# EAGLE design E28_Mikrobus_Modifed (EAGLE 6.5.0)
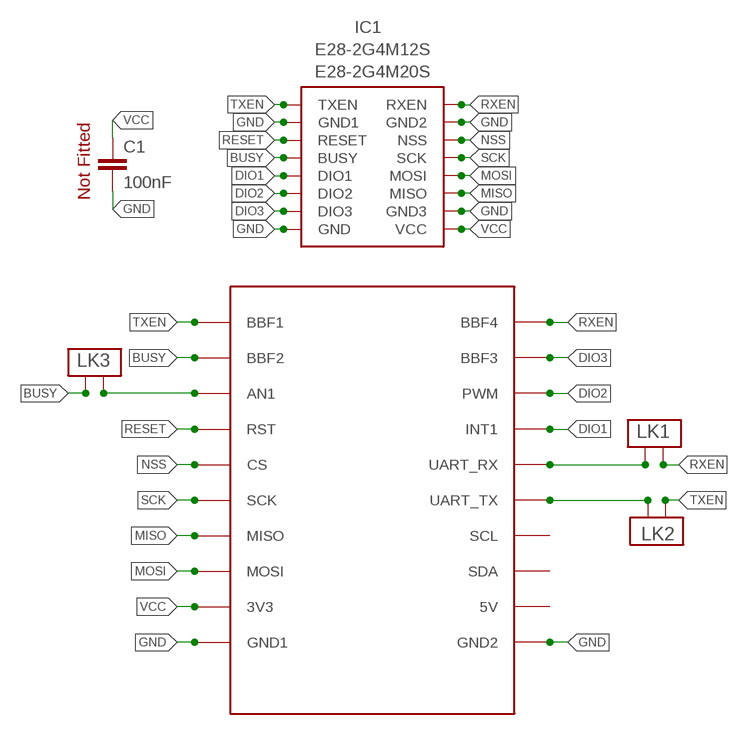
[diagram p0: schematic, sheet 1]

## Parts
C1  100nF  C-EUC0805  [C0805]
IC1  E28-2G4M12S  [E28-2G4M12S]
LK1  PCB_LINK  [PCB_LINK]
LK2  PCB_LINK  [PCB_LINK]
LK3  PCB_LINK  [PCB_LINK]
MB1  BBFRIENDY2  [PCB_SOCKET_BBFRIENDLY2]

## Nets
BUSY: IC1.BUSY LK3.P$2 MB1.BBF2
DIO1: IC1.DIO1 MB1.INT(INT1)
DIO2: IC1.DIO2 MB1.PWM
DIO3: IC1.DIO3 MB1.BBF3
GND [VDD]: C1.2 IC1.GND IC1.GND1 IC1.GND2 IC1.GND3 MB1.GND1(GND2) MB1.GND2(GND1)
MISO: IC1.MISO MB1.MISO
MOSI: IC1.MOSI MB1.MOSI
N$3: LK3.P$1 MB1.AN1
NSS: IC1.NSS MB1.CS
RESET: IC1.RESET MB1.RST
RXEN: IC1.RXEN LK1.P$1 MB1.BBF4
SCK: IC1.SCK MB1.SCK
TXEN: IC1.TXEN LK2.P$2 MB1.BBF1
UART_RX: LK1.P$2 MB1.RX(UART_RX)
UART_TX: LK2.P$1 MB1.TX(UART_TX)
VCC [VDD]: C1.1 IC1.VCC MB1.3V3
Unconnected: MB1.5V MB1.SCL MB1.SDA

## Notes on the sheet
- E28-2G4M20S
- Not Fitted

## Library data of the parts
C1 = resistor:C-EU: CAPACITOR, European symbol
IC1 = LMA2:E28-2G4M12S
LK1-LK3 = LMA2:PCB_LINK
MB1 = My_Mikrobus:BBFRIENDY2

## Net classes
0 default: width 0.152 mm
1 POWER: width 0.635 mm
2 VDD: width 0.635 mm

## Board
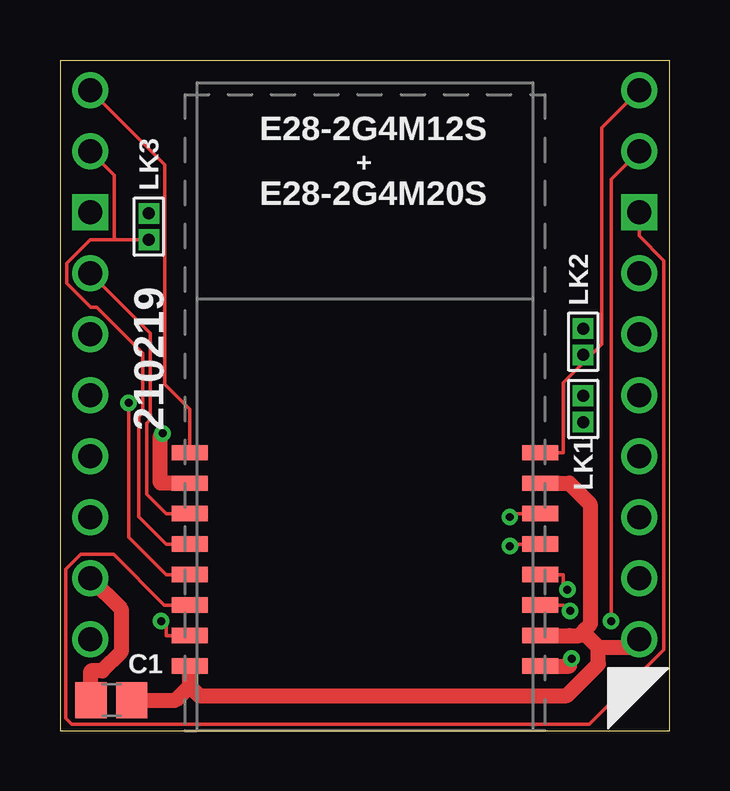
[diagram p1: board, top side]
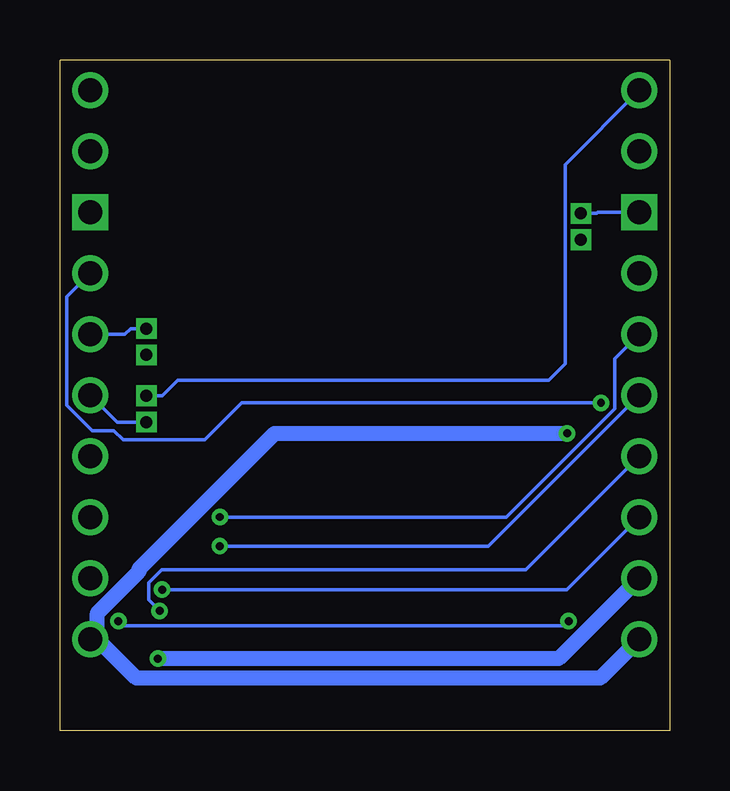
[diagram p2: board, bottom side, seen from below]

Size 25.4 x 27.94 mm. Coordinates in mm from the lower left corner, seen from the top.
Outline: 0,0 25.4,0 25.4,27.94 0,27.94 0,0
Copper layers (1*16): Top 0.0356mm / dielectric 1.5011mm / Bottom 0.0356mm
Design rules "LaenPCBOrder": minimum track width 6mil, minimum drill 13mil, track to track 6mil, track to pad 6mil, pad to pad 6mil, via to via 6mil, smd to smd 6mil, copper to edge 15mil, drill to drill 6mil, minimum pad ring 7mil, minimum via ring 7mil, stop-mask expansion 4mil, vias tented up to drill 0mil, thermal gap 10mil
tRestrict: area 4.6,15.4 to 20.9,28; area 6.5,1.9 to 19,15.4
bRestrict: area 4.6,15.4 to 20.9,27.9

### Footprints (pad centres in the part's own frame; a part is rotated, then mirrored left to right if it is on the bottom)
C0805 = smd 1.3 x 1.5: 1 -0.85,0; 2 0.85,0
E28-2G4M12S = smd 1.5 x 0.635: BUSY -7.3,7.77; DIO1 -7.3,6.5; DIO2 -7.3,5.23; DIO3 -7.3,3.96; GND -7.3,2.69; GND1 -7.3,10.31; GND2 7.3,10.31; GND3 7.3,3.96; MISO 7.3,5.23; MOSI 7.3,6.5; NSS 7.3,9.04; RESET -7.3,9.04; RXEN 7.3,11.58; SCK 7.3,7.77; TXEN -7.3,11.58; VCC 7.3,2.69
PCB_LINK = drill 0.5 pad 0.813 square: P$1 -0.55,0; P$2 0.55,0
PCB_SOCKET_BBFRIENDLY2 = drill 1: 3V3 -11.43,5.08; 5V 11.43,5.08; BBF1 -11.43,25.4; BBF2 -11.43,22.86; BBF3 11.43,22.86; BBF4 11.43,25.4; CS -11.43,15.24; GND1 -11.43,2.54; GND2 11.43,2.54; INT 11.43,17.78; MISO -11.43,10.16; MOSI -11.43,7.62; RST -11.43,17.78; RX 11.43,15.24; SCK -11.43,12.7; SCL 11.43,10.16; SDA 11.43,7.62; TX 11.43,12.7 | drill 1 square: AN1 -11.43,20.32; PWM 11.43,20.32

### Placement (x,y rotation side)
C1  2.14,1.27 0 top
IC1  12.7,0 0 top
LK1  21.8,16.2 90 top
LK2  21.8,13.4 90 top
LK3  3.7,21 270 top
MB1  12.7,1.27 0 top

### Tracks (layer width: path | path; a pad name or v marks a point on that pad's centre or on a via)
BUSY
  Top 0.152: IC1.BUSY 4.42,7.77 3.29,8.9 3.29,13.07 3.45,13.23 3.45,15.71 1.52,17.64 1.28,17.64 0.29,18.63 0.29,19.48 1.26,20.45 2.27,20.45 | 2.27,20.45 3.21,20.45 LK3.P$2 | MB1.BBF2 2.27,23.13 2.27,20.45
DIO1  (via drill 0.33 pad 0.69)
  Top 0.152: IC1.DIO1 4.42,6.5 2.86,8.06 v2.86,13.65
  Bottom 0.152: MB1.INT 25.11,18.07 25.11,13.55 24.05,12.5 23.15,12.5 22.77,12.12 19.36,12.12 17.83,13.65 v2.86,13.65
DIO2
  Top 0.152: MB1.PWM 24.13,20.61 25.16,19.58 25.16,3.37 22.06,0.27 0.49,0.27 0.24,0.51 0.24,6.71 0.86,7.34 2.24,7.34 4.35,5.23 IC1.DIO2
DIO3  (via drill 0.33 pad 0.69)
  Top 0.152: v22.97,4.56 22.97,22.97 MB1.BBF3 | v4.21,4.56 4.42,4.35 4.42,3.96 IC1.DIO3
  Bottom 0.152: v4.21,4.56 4.41,4.37 22.77,4.37 v22.97,4.56
GND  (via drill 0.33 pad 0.69)
  Top 0.635: 21.79,4.11 22.43,3.47 | 21.79,4.11 22.09,4.41 22.09,9.44 21.22,10.31 IC1.GND2 | 21.79,4.11 21.64,3.96 21.22,3.96 IC1.GND3 | 5.4,1.85 5.8,1.46 21.11,1.46 22.43,2.77 22.43,3.47 | 22.43,3.47 23.79,3.47 MB1.GND2 | IC1.GND1 4.18,10.31 4.18,12.29 v4.27,12.39 | C1.2 4.82,1.27 5.4,1.85 | 5.4,1.85 IC1.GND
  Bottom 0.635: MB1.GND1 2.9,2.18 22.22,2.18 23.85,3.81 | 23.85,3.81 MB1.GND2 | 23.85,3.81 23.85,4.89 22.12,6.63 22.12,6.72 16.45,12.39 v4.27,12.39
MISO  (via drill 0.33 pad 0.69)
  Top 0.152: v21.25,4.99 21.22,4.99 20.98,5.23 IC1.MISO
  Bottom 0.152: MB1.MISO 6,6.7 21.16,6.7 21.71,6.16 21.71,5.45 v21.25,4.99
MOSI  (via drill 0.33 pad 0.69)
  Top 0.152: IC1.MOSI 20.98,6.5 20.98,6.03 v21.14,5.87
  Bottom 0.152: MB1.MOSI 4.29,5.87 v21.14,5.87
N$3
  Bottom 0.152: LK3.P$1 3.04,21.55 3,21.59 MB1.AN1
NSS  (via drill 0.33 pad 0.69)
  Top 0.152: IC1.NSS 19.02,9.04 18.88,8.9 v18.74,8.9
  Bottom 0.152: v18.74,8.9 6.81,8.9 2.29,13.42 2.29,15.49 MB1.CS
RESET
  Top 0.152: MB1.RST 3.77,16.55 3.77,12.96 3.6,12.8 3.6,9.86 4.42,9.04 IC1.RESET
RXEN
  Top 0.152: MB1.BBF4 22.57,25.11 22.57,16.09 22.13,15.65 | IC1.RXEN 20.98,11.58 20.98,14.5 22.13,15.65 | LK1.P$1 22.13,15.65
SCK  (via drill 0.33 pad 0.69)
  Top 0.152: IC1.SCK 19.02,7.77 18.93,7.68 v18.74,7.68
  Bottom 0.152: v18.74,7.68 7.56,7.68 MB1.SCK
TXEN
  Top 0.152: MB1.BBF1 4.36,23.58 4.36,14.43 5.4,13.39 IC1.TXEN
  Bottom 0.152: LK2.P$2 21.14,13.95 20.49,14.61 5.04,14.61 4.36,15.29 4.36,23.58 MB1.BBF1
UART_RX
  Bottom 0.152: LK1.P$2 22.46,16.75 22.7,16.51 MB1.RX
UART_TX
  Bottom 0.152: MB1.TX 23.01,12.85 LK2.P$1
VCC  (via drill 0.33 pad 0.69)
  Top 0.635: v21.32,3 21.22,2.9 21.22,2.69 IC1.VCC | C1.1 1.29,2.49 1.77,2.49 2.54,3.27 2.54,5.08 MB1.3V3
  Bottom 0.635: MB1.3V3 4.62,3 v21.32,3

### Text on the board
tNames: E28-2G4M12S | + | E28-2G4M20S | LK3 | LK2 | 210219 | LK1 | C1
